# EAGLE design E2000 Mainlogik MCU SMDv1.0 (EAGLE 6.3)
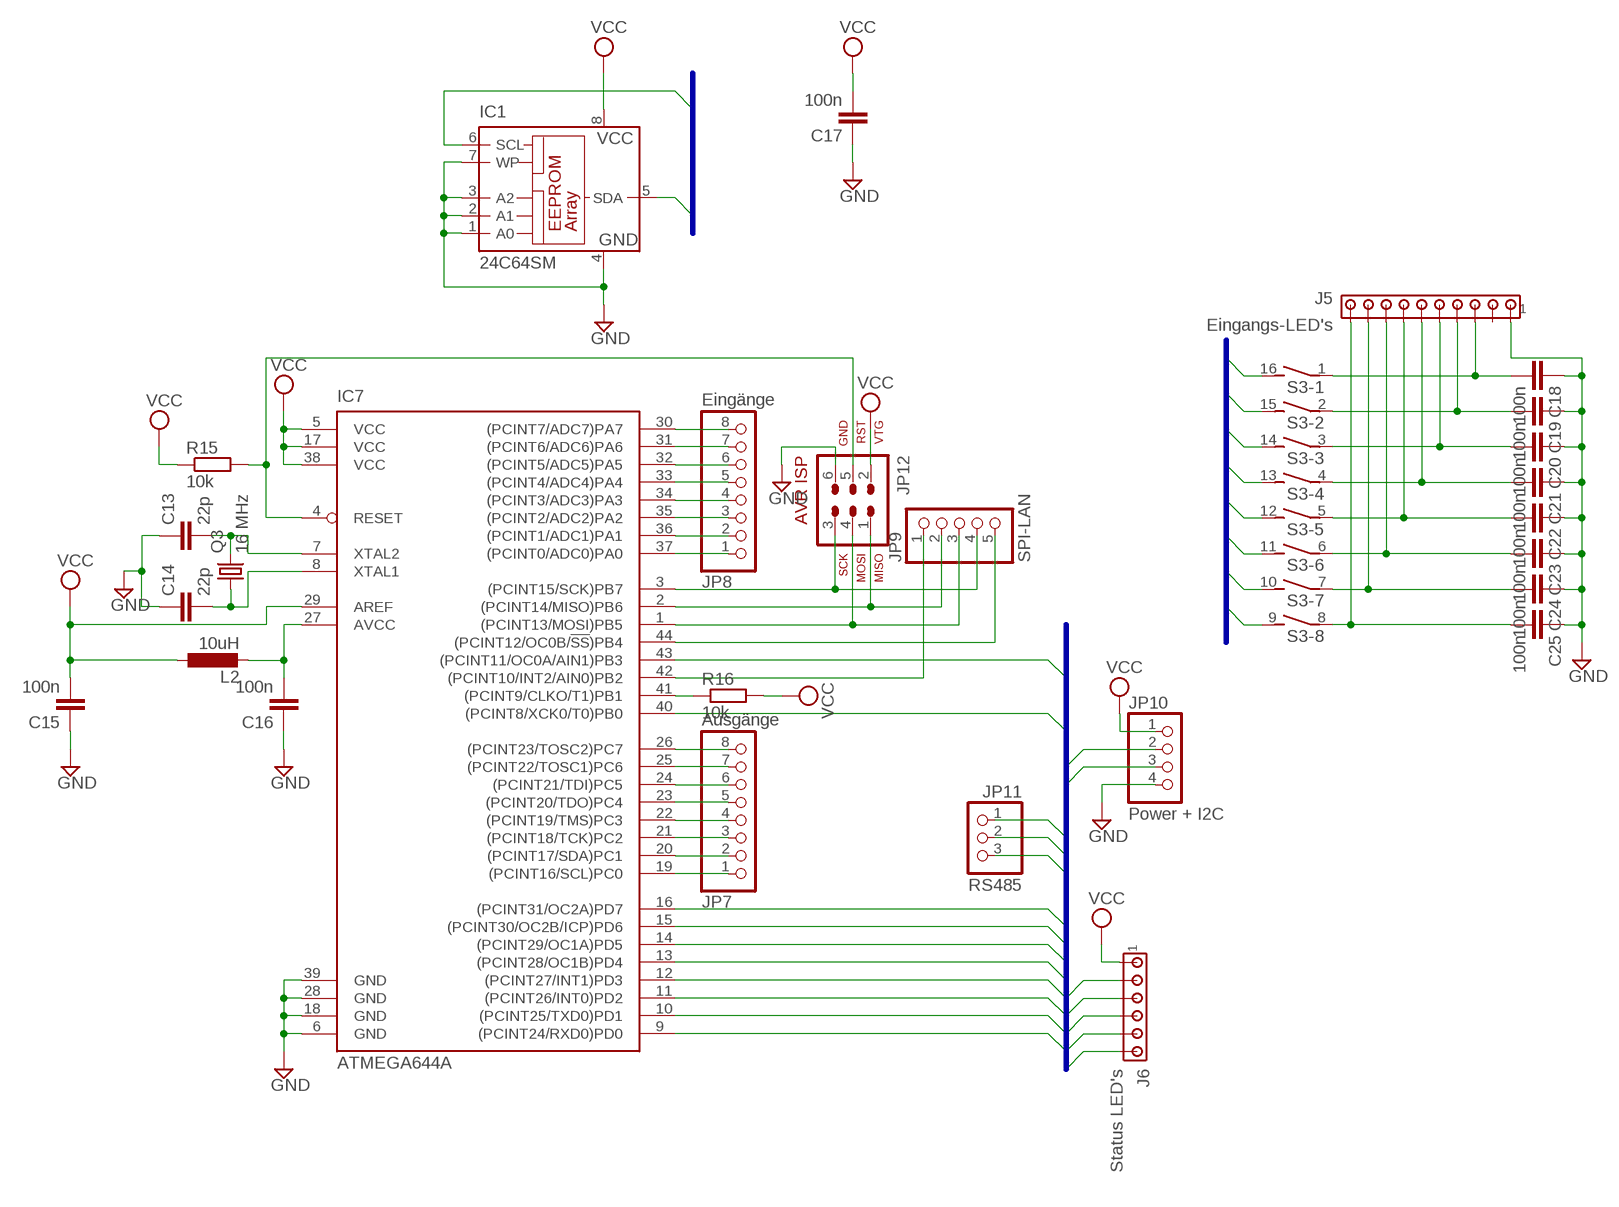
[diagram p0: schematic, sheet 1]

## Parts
C13  22p  C-EUC1206  [C1206]
C14  22p  C-EUC1206  [C1206]
C15  100n  C-EUC1206  [C1206]
C16  100n  C-EUC1206  [C1206]
C17  100n  C-EUC1206  [C1206]
C18  100n  C-EUC1206  [C1206]
C19  100n  C-EUC1206  [C1206]
C20  100n  C-EUC1206  [C1206]
C21  100n  C-EUC1206  [C1206]
C22  100n  C-EUC1206  [C1206]
C23  100n  C-EUC1206  [C1206]
C24  100n  C-EUC1206  [C1206]
C25  100n  C-EUC1206  [C1206]
IC1  24C64SM  [SO-08M]
IC7  ATMEGA644A  [TQFP44]
J5  Eingangs-LED's  MTA10-100  [10X10MTA]
J6  Status LED's  MTA06-100  [10X06MTA]
JP7  Ausgänge  PINHD-1X8_2.54-SMD  [1X08SMD]
JP8  Eingänge  PINHD-1X8_2.54-SMD  [1X08SMD]
JP9  SPI-LAN  PINHD-1X5_2.54-SMD  [1X05SMD]
JP10  Power + I2C  PINHD-1X4_2.54-SMD  [1X04SMD]
JP11  RS485  PINHD-1X3_2.54-SMD  [1X03SMD]
JP12  AVR-ISP-6  [AVR-ISP-6]
L2  10uH  L-EUL1206  [C1206]
Q3  16 MHz  CRYSTALHC49S  [HC49/S]
R15  10k  R-EU_0207/10  [0207/10]
R16  10k  R-EU_0207/10  [0207/10]
S3  DIP08S  [DIP08S]

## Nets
A1: IC7.19((PCINT16/SCL)PC0) JP7.1
A2: IC7.20((PCINT17/SDA)PC1) JP7.2
A3: IC7.21((PCINT18/TCK)PC2) JP7.3
A4: IC7.22((PCINT19/TMS)PC3) JP7.4
A5: IC7.23((PCINT20/TDO)PC4) JP7.5
A6: IC7.24((PCINT21/TDI)PC5) JP7.6
A7: IC7.25((PCINT22/TOSC1)PC6) JP7.7
A8: IC7.26((PCINT23/TOSC2)PC7) JP7.8
CS: IC7.44((PCINT12/OC0B/!SS!)PB4) JP9.5
E1: IC7.37((PCINT0/ADC0)PA0) JP8.1 S3.16
E2: IC7.36((PCINT1/ADC1)PA1) JP8.2 S3.15
E3: IC7.35((PCINT2/ADC2)PA2) JP8.3 S3.14
E4: IC7.34((PCINT3/ADC3)PA3) JP8.4 S3.13
E5: IC7.33((PCINT4/ADC4)PA4) JP8.5 S3.12
E6: IC7.32((PCINT5/ADC5)PA5) JP8.6 S3.11
E7: IC7.31((PCINT6/ADC6)PA6) JP8.7 S3.10
E8: IC7.30((PCINT7/ADC7)PA7) JP8.8 S3.9
EXT3: IC7.13((PCINT28/OC1B)PD4) JP11.2
EXT4: IC7.14((PCINT29/OC1A)PD5) J6.1
EXT5: IC7.15((PCINT30/OC2B/ICP)PD6) J6.2
EXT6: IC7.16((PCINT31/OC2A)PD7) J6.3
EXT7: IC7.40((PCINT8/XCK0/T0)PB0) J6.4
EXT8: IC7.43((PCINT11/OC0A/AIN1)PB3) J6.5
GND: C13.1 C14.1 C15.1 C16.1 C17.1 C18.1 C19.1 C20.1 C21.1 C22.1 C23.1 C24.1 C25.1 IC1.1(A0) IC1.2(A1) IC1.3(A2) IC1.4(GND) IC1.7(WP) IC7.6(GND) IC7.18(GND) IC7.28(GND) IC7.39(GND) J5.1 JP10.4 JP12.6
INT: IC7.42((PCINT10/INT2/AIN0)PB2) JP9.1
MISO: IC7.2((PCINT14/MISO)PB6) JP9.2 JP12.1
MOSI: IC7.1((PCINT13/MOSI)PB5) JP9.3 JP12.4
N$1: C18.2 J5.3 S3.1
N$2: C19.2 J5.4 S3.2
N$3: IC7.41((PCINT9/CLKO/T1)PB1) R16.1
N$4: C20.2 J5.5 S3.3
N$5: C21.2 J5.6 S3.4
N$6: C22.2 J5.7 S3.5
N$7: C23.2 J5.8 S3.6
N$8: C24.2 J5.9 S3.7
N$9: C25.2 J5.10 S3.8
N$17: C14.2 IC7.8(XTAL1) Q3.1
N$18: C13.2 IC7.7(XTAL2) Q3.2
N$19: C16.2 IC7.27(AVCC) L2.2
RST: IC7.4(RESET) JP12.5 R15.2
RX: IC7.9((PCINT24/RXD0)PD0) JP11.3
SCK: IC7.3((PCINT15/SCK)PB7) JP9.4 JP12.3
SCL: IC1.6(SCL) IC7.11((PCINT26/INT0)PD2) JP10.2
SDA: IC1.5(SDA) IC7.12((PCINT27/INT1)PD3) JP10.3
TX: IC7.10((PCINT25/TXD0)PD1) JP11.1
VCC: C15.2 C17.2 IC1.8(VCC) IC7.5(VCC) IC7.17(VCC) IC7.29(AREF) IC7.38(VCC) J6.6 JP10.1 JP12.2 L2.1 R15.1 R16.2
Unconnected: J5.2

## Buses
E1,E2,E3,E4,E5,E6,E7,E8
RX,TX,SCL,SDA,EXT3,EXT4,EXT5,EXT6,EXT7,EXT8
SCL,SDA

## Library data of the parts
C13-C25 = rcl:C-EU: CAPACITOR, European symbol
IC1 = microchip:24*: Serial EEPROM I2C; MF: RAMTRON INTERNATIONAL CORP; MPN: FM24C64-S; OC_FARNELL: 9882685; OC_NEWARK: 98H0189
IC7 = atmel:ATMEGA644: 8-bit Microcontroller with 64K Bytes In-System Programmable Flash Source: http://www.atmel.com/dyn/resources/prod_documents/doc2593.pdf; MPN: ATMEGA644PV-10AU; OC_FARNELL: 1455123; OC_NEWARK: 58M3748
J5 = con-amp:MTA10-100: AMP connector
J6 = con-amp:MTA06-100: AMP connector
JP7 JP8 = pinhead:PINHD-1X8: PIN HEADER
JP9 = pinhead:PINHD-1X5: PIN HEADER
JP10 = pinhead:PINHD-1X4: PIN HEADER
JP11 = pinhead:PINHD-1X3: PIN HEADER
JP12 = avr-6:AVR-ISP-6: AVR ISP-6 Serial Programming Header
L2 = rcl:L-EU: INDUCTOR, European symbol
Q3 = crystal:CRYSTAL: CRYSTAL; OC_FARNELL: 1667008; OC_NEWARK: unknown
R15 R16 = rcl:R-EU_: RESISTOR, European symbol
S3 = switch-dil:DIP08S: DIL/CODE SWITCH; OC_FARNELL: unknown; OC_NEWARK: unknown

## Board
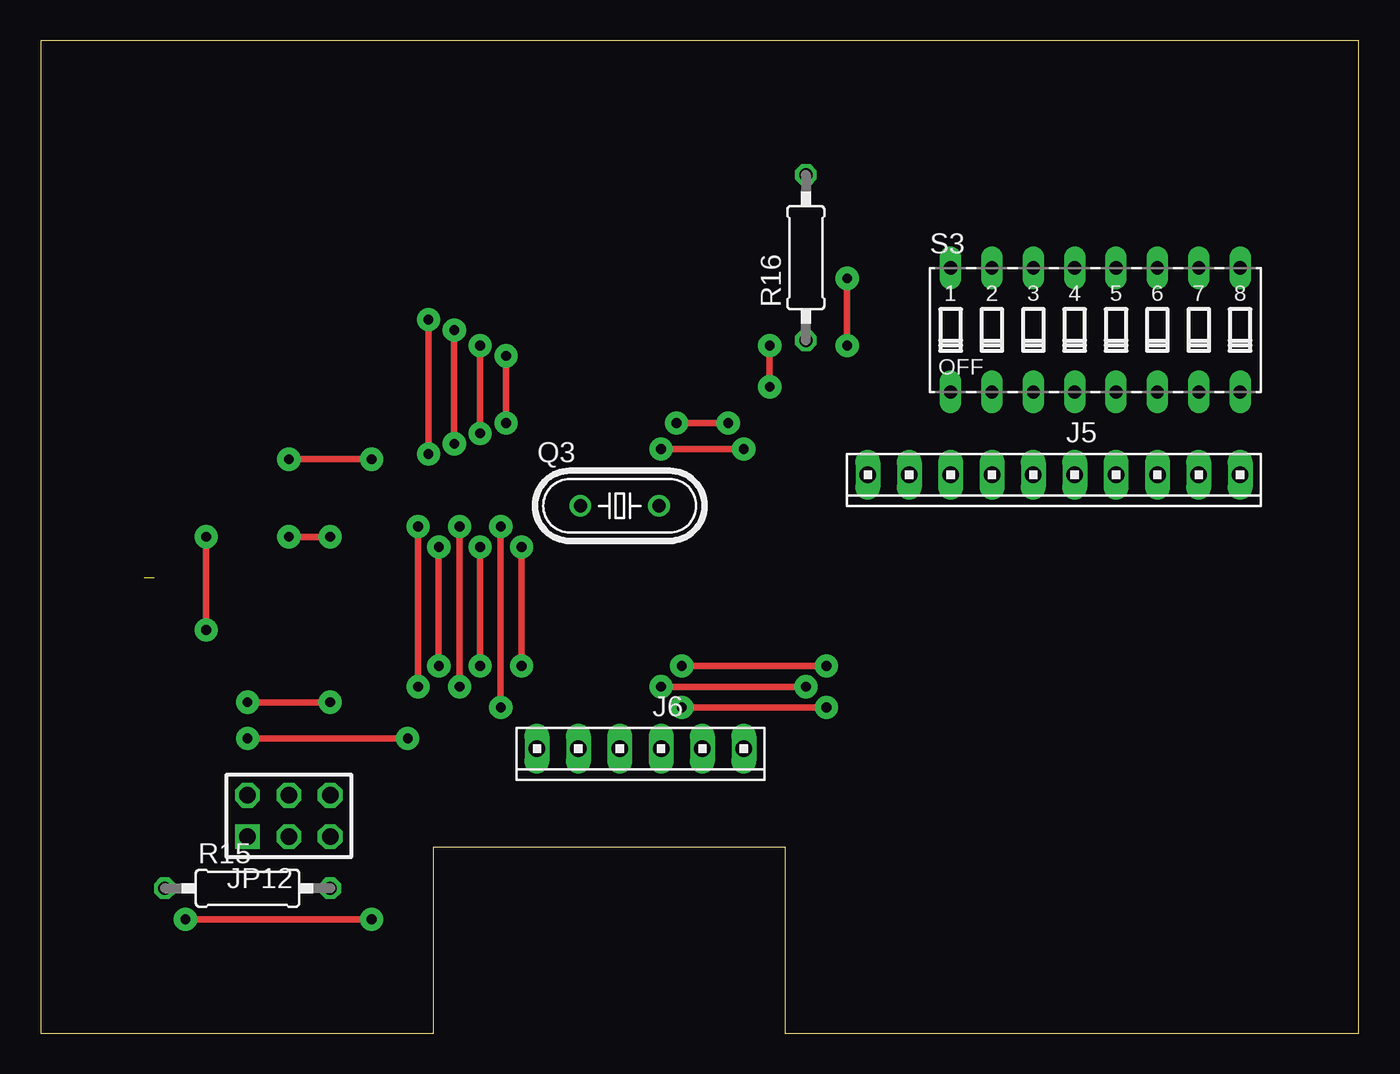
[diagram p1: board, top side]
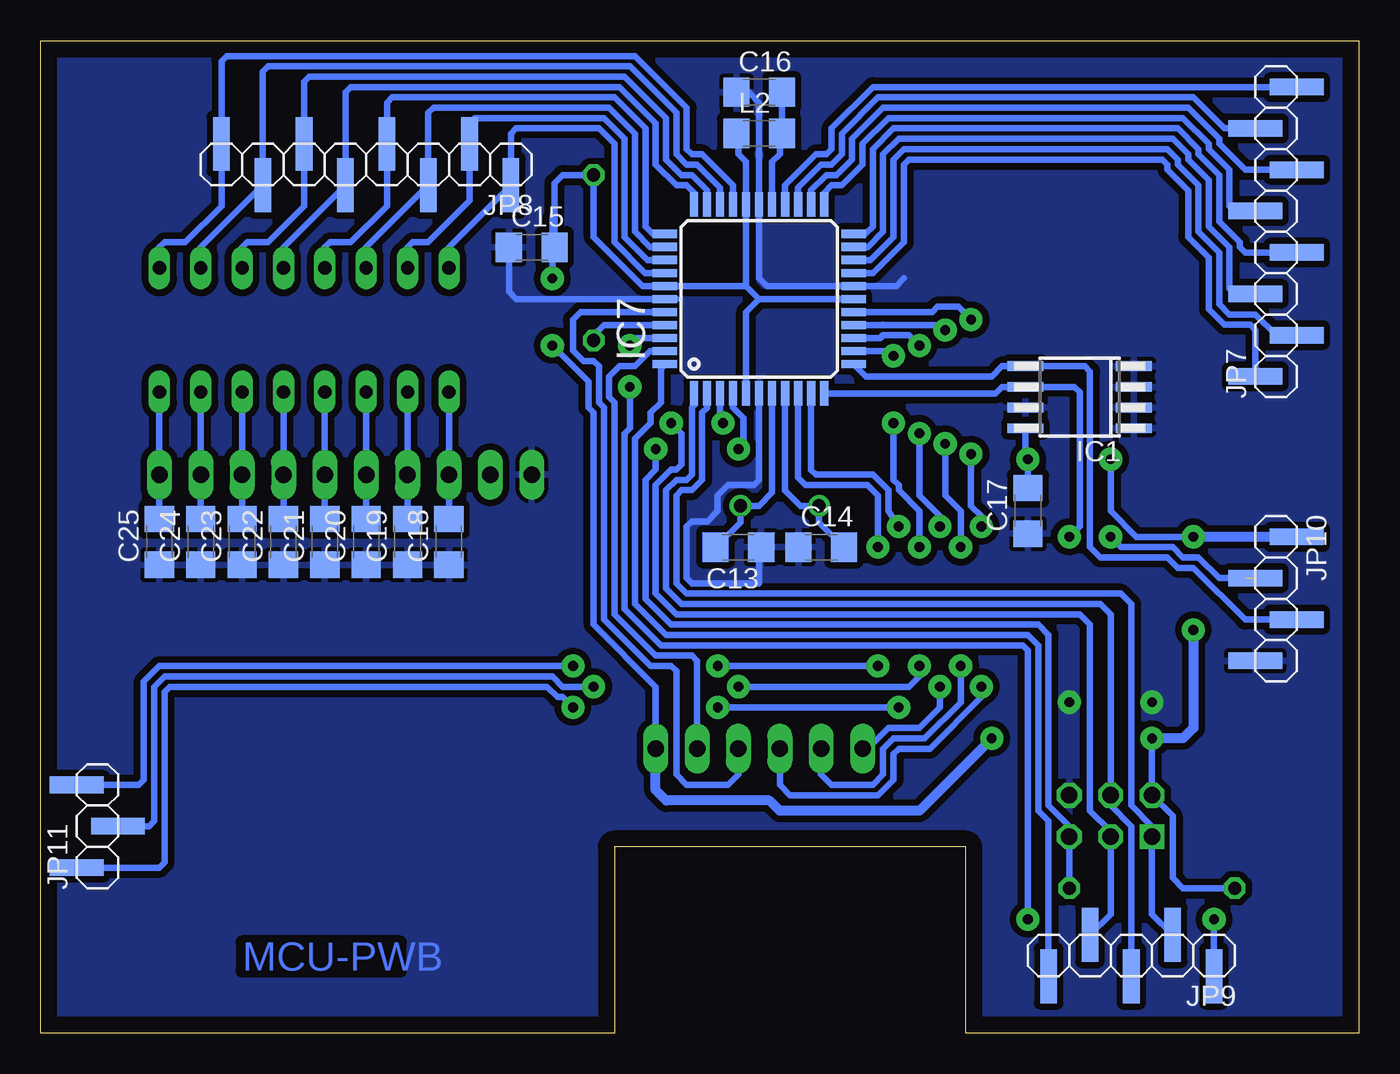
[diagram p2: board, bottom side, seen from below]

Size 80.95 x 60.95 mm. Coordinates in mm from the lower left corner, seen from the top.
Outline: 0,0 24.13,0 24.13,11.43 45.72,11.43 45.72,0 80.95,0 80.95,60.95 0,60.95 0,0
Copper layers (1*16): Top 0.035mm / dielectric 1.5mm / Bottom 0.035mm
Design rules "default": minimum track width 10mil, minimum drill 24mil, track to track 8mil, track to pad 8mil, pad to pad 8mil, via to via 8mil, smd to smd 8mil, copper to edge 40mil, drill to drill 8mil, minimum pad ring 10mil, minimum via ring 8mil, stop-mask expansion 4mil, vias tented up to drill 0mil, thermal gap 10mil

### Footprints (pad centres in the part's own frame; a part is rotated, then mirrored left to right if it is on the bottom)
C1206 = smd 1.6 x 1.8: 1 -1.4,0; 2 1.4,0
SO-08M = smd 0.6 x 2.2: 1 -1.905,-3.33; 2 -0.635,-3.33; 3 0.635,-3.33; 4 1.905,-3.33; 5 1.905,3.33; 6 0.635,3.33; 7 -0.635,3.33; 8 -1.905,3.33
TQFP44 = smd 1.5 x 0.5: 1 -5.8,4; 2 -5.8,3.2; 3 -5.8,2.4; 4 -5.8,1.6; 5 -5.8,0.8; 6 -5.8,0; 7 -5.8,-0.8; 8 -5.8,-1.6; 9 -5.8,-2.4; 10 -5.8,-3.2; 11 -5.8,-4; 23 5.8,-4; 24 5.8,-3.2; 25 5.8,-2.4; 26 5.8,-1.6; 27 5.8,-0.8; 28 5.8,0; 29 5.8,0.8; 30 5.8,1.6; 31 5.8,2.4; 32 5.8,3.2; 33 5.8,4 | smd 0.5 x 1.5: 12 -4,-5.8; 13 -3.2,-5.8; 14 -2.4,-5.8; 15 -1.6,-5.8; 16 -0.8,-5.8; 17 0,-5.8; 18 0.8,-5.8; 19 1.6,-5.8; 20 2.4,-5.8; 21 3.2,-5.8; 22 4,-5.8; 34 4,5.8; 35 3.2,5.8; 36 2.4,5.8; 37 1.6,5.8; 38 0.8,5.8; 39 0,5.8; 40 -0.8,5.8; 41 -1.6,5.8; 42 -2.4,5.8; 43 -3.2,5.8; 44 -4,5.8
10X10MTA = drill 1.016 long: 1 11.43,0; 2 8.89,0; 3 6.35,0; 4 3.81,0; 5 1.27,0; 6 -1.27,0; 7 -3.81,0; 8 -6.35,0; 9 -8.89,0; 10 -11.43,0
10X06MTA = drill 1.016 long: 1 6.35,0; 2 3.81,0; 3 1.27,0; 4 -1.27,0; 5 -3.81,0; 6 -6.35,0
1X08SMD = smd 1.016 x 3.302: 1 -1.27,1.27; 2 1.27,-1.27; 3 3.81,1.27; 4 6.35,-1.27; 5 8.89,1.27; 6 11.43,-1.27; 7 13.97,1.27; 8 16.51,-1.27
1X05SMD = smd 1.016 x 3.302: 1 -1.27,1.27; 2 1.27,-1.27; 3 3.81,1.27; 4 6.35,-1.27; 5 8.89,1.27
1X04SMD = smd 1.016 x 3.302: 1 -1.27,1.27; 2 1.27,-1.27; 3 3.81,1.27; 4 6.35,-1.27
1X03SMD = smd 1.016 x 3.302: 1 -1.27,1.27; 2 1.27,-1.27; 3 3.81,1.27
AVR-ISP-6 = drill 1.016 square: 1 -2.54,-1.27 | drill 1.016 octagon: 2 -2.54,1.27; 3 0,-1.27; 4 0,1.27; 5 2.54,-1.27; 6 2.54,1.27
HC49/S = drill 0.813: 1 -2.413,0; 2 2.413,0
0207/10 = drill 0.813 octagon: 1 -5.08,0; 2 5.08,0
DIP08S = drill 0.813 long: 1 -8.89,-3.81; 2 -6.35,-3.81; 3 -3.81,-3.81; 4 -1.27,-3.81; 5 1.27,-3.81; 6 3.81,-3.81; 7 6.35,-3.81; 8 8.89,-3.81; 9 8.89,3.81; 10 6.35,3.81; 11 3.81,3.81; 12 1.27,3.81; 13 -1.27,3.81; 14 -3.81,3.81; 15 -6.35,3.81; 16 -8.89,3.81

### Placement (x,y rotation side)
C13  38.1,29.84 180 bottom
C14  33.02,29.84 0 bottom
C15  50.8,48.26 0 bottom
C16  36.83,57.78 0 bottom
C17  20.32,32.07 90 bottom
C18  55.88,30.16 90 bottom
C19  58.42,30.16 90 bottom
C20  60.96,30.16 90 bottom
C21  63.5,30.16 90 bottom
C22  66.04,30.16 90 bottom
C23  68.58,30.16 90 bottom
C24  71.12,30.16 90 bottom
C25  73.66,30.16 90 bottom
IC1  17.14,39.05 90 bottom
IC7  36.83,45.09 90 bottom
J5  62.23,34.29 180 top
J6  36.83,17.46 180 top
JP7  5.08,41.59 90 bottom
JP8  53.34,53.34 180 bottom
JP9  10.16,4.76 180 bottom
JP10  5.08,29.21 270 bottom
JP11  77.47,11.43 90 bottom
JP12  15.24,13.34 0 top
L2  36.83,55.24 0 bottom
Q3  35.56,32.38 0 top
R15  12.7,8.89 0 top
R16  46.99,47.62 90 top
S3  64.77,43.18 0 top

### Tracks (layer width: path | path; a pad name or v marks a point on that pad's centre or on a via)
A1
  Bottom 0.406: IC7.19 29.83,46.69 27.94,48.58 27.94,53.34 27.62,53.66 12.07,53.66 11.75,53.34 11.75,53.02 10.48,51.75 10.48,48.9 9.21,47.62 9.21,44.45 8.26,43.5 6.67,43.5 6.35,43.18 JP7.1
A2
  Bottom 0.406: IC7.20 29.98,47.48 28.57,48.9 28.57,53.66 27.94,54.29 11.75,54.29 11.11,53.66 11.11,53.34 9.84,52.07 9.84,49.21 8.57,47.94 8.57,44.77 7.94,44.13 6.35,44.13 5.08,42.86 JP7.2
A3
  Bottom 0.406: IC7.21 30.14,48.28 29.21,49.21 29.21,53.98 28.26,54.93 11.43,54.93 10.48,53.98 10.48,53.66 9.21,52.39 9.21,49.53 7.94,48.26 7.94,45.72 7.62,45.4 JP7.3
A4
  Bottom 0.406: IC7.22 30.29,49.09 29.84,49.53 29.84,54.29 28.57,55.56 11.11,55.56 9.84,54.29 9.84,53.98 8.57,52.7 8.57,49.85 7.3,48.58 7.3,48.26 6.99,47.94 JP7.4
A5
  Bottom 0.406: IC7.23 32.83,51.62 32.38,52.07 31.75,52.07 30.48,53.34 30.48,54.61 28.89,56.2 10.79,56.2 9.21,54.61 9.21,54.29 7.94,53.02 7.94,50.8 7.62,50.48 JP7.5
A6
  Bottom 0.406: IC7.24 33.63,51.78 32.7,52.7 32.07,52.7 31.11,53.66 31.11,54.93 29.21,56.83 10.48,56.83 8.57,54.93 8.57,54.61 6.99,53.02 JP7.6
A7
  Bottom 0.406: IC7.25 34.43,51.93 33.02,53.34 32.38,53.34 31.75,53.98 31.75,55.24 29.53,57.47 10.16,57.47 8.26,55.56 JP7.7
A8
  Bottom 0.406: IC7.26 35.23,52.08 33.34,53.98 32.7,53.98 32.38,54.29 32.38,55.56 29.84,58.1 JP7.8
CS
  Bottom 0.406: IC7.44 42.86,40.85 42.86,38.73 43.5,38.1 43.5,37.47 44.45,36.51 44.45,26.35 42.54,24.45 20.32,24.45 19.68,23.81 19.68,13.65 19.05,13.02 JP9.5
E1
  Bottom 0.406: IC7.37 43.83,46.69 45.72,48.58 45.72,54.61 46.67,55.56 51.75,55.56 52.07,55.24 JP8.1 55.88,48.26 S3.16
E2
  Bottom 0.406: IC7.36 43.67,47.48 45.08,48.9 45.08,54.93 46.35,56.2 54.29,56.2 54.61,55.88 JP8.2 54.61,51.12 57.15,48.58 58.1,48.58 58.42,48.26 S3.15
E3
  Bottom 0.406: IC7.35 43.52,48.28 44.45,49.21 44.45,55.24 46.04,56.83 56.83,56.83 57.15,56.52 JP8.3 60.96,48.26 S3.14
E4
  Bottom 0.406: IC7.34 43.37,49.09 43.81,49.53 43.81,55.56 45.72,57.47 59.37,57.47 59.69,57.15 JP8.4 59.69,50.8 61.91,48.58 63.18,48.58 63.5,48.26 S3.13
E5
  Bottom 0.406: IC7.33 40.83,51.62 41.27,52.07 41.91,52.07 43.18,53.34 43.18,55.88 45.4,58.1 61.91,58.1 62.23,57.78 JP8.5 66.04,48.26 S3.12
E6
  Bottom 0.406: IC7.32 40.03,51.78 40.96,52.7 41.59,52.7 42.54,53.66 42.54,56.2 45.08,58.74 64.45,58.74 64.77,58.42 JP8.6 64.77,50.8 66.99,48.58 68.26,48.58 68.58,48.26 S3.11
E7
  Bottom 0.406: IC7.31 39.23,51.93 40.64,53.34 41.27,53.34 41.91,53.98 41.91,56.52 44.77,59.37 66.99,59.37 67.31,59.05 JP8.7 71.12,48.26 S3.10
E8
  Bottom 0.406: IC7.30 38.43,52.08 40.32,53.98 40.96,53.98 41.27,54.29 41.27,56.83 44.45,60.01 69.53,60.01 69.85,59.69 JP8.8 69.85,50.8 72.07,48.58 73.34,48.58 73.66,48.26 S3.9
EXT3  (via drill 0.6 pad 1.42)
  Top 0.406: v28.57,41.59 v28.57,37.47 | v46.99,21.27 v38.1,21.27 | v26.99,22.54 v26.99,29.84
  Bottom 0.406: IC7.13 28.87,41.88 v28.57,41.59 | v46.99,21.27 48.89,21.27 49.53,21.91 73.34,21.91 73.98,21.27 73.98,13.02 74.3,12.7 JP11.2 | v38.1,21.27 27.62,21.27 26.99,21.91 v26.99,22.54 | v26.99,29.84 26.99,32.07 28.26,33.34 28.26,33.66 28.57,33.97 v28.57,37.47
EXT4  (via drill 0.6 pad 1.42)
  Top 0.406: v26.99,42.23 v26.99,36.83 | v25.72,31.11 v25.72,21.27
  Bottom 0.406: v26.99,42.23 27.62,42.86 29.21,42.86 29.39,42.69 IC7.14 | v26.99,36.83 26.99,33.02 25.72,31.75 v25.72,31.11 | v25.72,21.27 25.72,20 26.99,18.73 28.89,18.73 30.16,17.46 J6.1
EXT5  (via drill 0.6 pad 1.42)
  Top 0.406: v25.4,43.18 v25.4,36.2 | v24.45,29.84 v24.45,22.54
  Bottom 0.406: v25.4,43.18 25.71,43.48 29.2,43.48 29.21,43.5 29.22,43.48 IC7.15 | v25.4,36.2 25.4,33.02 24.45,32.07 v24.45,29.84 | v24.45,22.54 24.45,20.32 26.67,18.1 28.57,18.1 29.21,17.46 29.21,15.88 29.84,15.24 32.38,15.24 33.02,15.88 J6.2
EXT6  (via drill 0.6 pad 1.42)
  Top 0.406: v23.81,43.81 v23.81,35.56 | v23.18,31.11 v23.18,21.27
  Bottom 0.406: v23.81,43.81 24.6,44.6 25.88,44.6 26.2,44.28 IC7.16 | v23.81,35.56 23.81,32.38 23.18,31.75 v23.18,31.11 | v23.18,21.27 23.18,20.64 26.35,17.46 28.26,17.46 28.57,17.14 28.57,15.56 29.53,14.61 34.92,14.61 35.56,15.24 J6.3
EXT7
  Bottom 0.406: IC7.40 47.79,44.28 48.26,43.81 48.26,41.91 47.62,41.27 46.99,41.27 46.67,40.96 46.67,38.73 46.35,38.42 46.35,25.4 43.5,22.54 42.23,22.54 41.91,22.23 41.91,15.88 41.27,15.24 38.73,15.24 38.1,15.88 J6.4
EXT8
  Bottom 0.406: IC7.43 43.52,41.88 44.45,40.96 45.4,40.96 46.04,40.32 46.04,39.05 45.72,38.73 45.72,25.72 43.18,23.18 40.96,23.18 40.64,22.86 J6.5
GND  (via drill 0.6 pad 1.42)
  Top 0.406: v17.78,20.32 v12.7,20.32
  Bottom 0.406: 37.46,57.78 36.83,57.15 IC7.28 36.83,46.35 36.36,45.88 IC7.18 28.41,45.88 27.94,46.35 | 41.91,45.09 IC7.39 51.75,45.09 52.2,45.53 C15.1 | IC7.6 36.83,33.97 37.15,33.66 38.73,33.66 39.37,33.02 39.37,32.07 40,31.43 40.96,31.43 41.27,31.11 41.27,27.94 40.96,27.62 36.83,27.62 36.83,29.71 C13.1
  pour Bottom (isolate 0.406): -1.27,62.23 82.55,62.23 82.55,-1.27 44.45,-1.27 44.45,10.16 25.4,10.16 25.4,-1.27 -1.27,-1.27
INT  (via drill 0.6 pad 1.42)
  Top 0.406: v44.77,42.23 v44.77,39.69 | v8.89,6.99 v20.32,6.99
  Bottom 0.406: v20.32,6.99 20.32,23.5 20.64,23.81 42.86,23.81 45.08,26.04 45.08,36.83 44.77,37.15 v44.77,39.69 | IC7.42 44.31,42.69 v44.77,42.23 | JP9.1 v8.89,6.99
MISO
  Bottom 0.406: IC7.2 40.03,38.39 40.32,38.1 40.32,33.97 40.96,33.34 41.59,33.34 41.91,33.02 41.91,27.62 41.27,26.99 14.61,26.99 13.97,26.35 13.97,13.97 12.7,12.7 JP12.1 12.7,7.3 JP9.2
MOSI
  Bottom 0.406: IC7.1 40.83,38.55 40.96,38.42 40.96,34.29 41.27,33.97 41.91,33.97 42.54,33.34 42.54,27.3 41.59,26.35 15.88,26.35 15.24,25.72 JP12.4 15.24,13.97 13.97,12.7 JP9.3
N$1
  Bottom 0.406: C18.2 J5.3 S3.1
N$2
  Bottom 0.406: C19.2 J5.4 S3.2
N$3
  Bottom 0.406: IC7.41 46.37,43.48 46.99,42.86 R16.1
N$4
  Bottom 0.406: C20.2 J5.5 S3.3
N$5
  Bottom 0.406: C21.2 J5.6 S3.4
N$6
  Bottom 0.406: C22.2 J5.7 S3.5
N$7
  Bottom 0.406: C23.2 J5.8 S3.6
N$8
  Bottom 0.406: S3.7 J5.9 C24.2
N$9
  Bottom 0.406: C25.2 J5.10 S3.8
N$17
  Bottom 0.406: IC7.8 35.23,33.33 34.29,32.38 Q3.1 33.15,31.37 C14.2
N$18
  Bottom 0.406: IC7.7 36.03,33.19 36.83,32.38 Q3.2 37.97,31.37 C13.2
N$19
  Bottom 0.406: IC7.27 36.03,53.51 35.56,53.98 35.56,55.12 L2.2 C16.2
RST  (via drill 0.6 pad 1.42)
  Top 0.406: v38.1,35.88 v43.18,35.88
  Bottom 0.406: R15.2 JP12.5 17.78,12.7 19.05,13.97 19.05,24.45 19.68,25.08 42.23,25.08 43.81,26.67 43.81,33.97 43.18,34.61 v43.18,35.88 | IC7.4 38.43,38.43 37.78,37.78 37.78,36.2 v38.1,35.88
RX  (via drill 0.6 pad 1.42)
  Top 0.406: v29.53,29.84 v29.53,22.54 | v48.26,22.54 v39.37,22.54
  Bottom 0.406: IC7.9 34.43,34.11 33.97,33.66 30.16,33.66 29.53,33.02 v29.53,29.84 | v48.26,22.54 73.66,22.54 74.61,21.59 74.61,15.56 74.93,15.24 JP11.3 | v39.37,22.54 v29.53,22.54
SCK  (via drill 0.6 pad 1.42)
  Top 0.406: v39.05,37.47 v42.23,37.47
  Bottom 0.406: IC7.3 39.23,37.6 v39.05,37.47 | v42.23,37.47 41.59,36.83 41.59,34.92 41.91,34.61 42.23,34.61 43.18,33.66 43.18,26.99 41.91,25.72 17.14,25.72 16.51,25.08 16.51,13.65 15.24,12.38 JP12.3 15.24,7.3 JP9.4
SCL  (via drill 0.6 pad 1.42)  (1 unrouted)
  Top 0.406: v15.24,30.48 v17.78,30.48
  Bottom 0.406: IC7.11 22.31,39.28 21.91,39.69 IC1.6 17.46,39.69 17.14,39.37 17.14,31.11 v17.78,30.48 | 7.3,27.62 6.99,27.94 | JP10.2 8.57,27.94 9.84,29.21 10.79,29.21 11.43,29.84 14.61,29.84 v15.24,30.48
SDA
  Bottom 0.406: IC7.12 30.27,40.32 22.54,40.32 21.91,40.96 IC1.5 16.83,40.96 16.51,40.64 16.51,29.84 15.88,29.21 11.75,29.21 11.11,28.57 10.16,28.57 6.99,25.4 JP10.3
TX  (via drill 0.6 pad 1.42)
  Top 0.406: v48.26,20 v39.37,20 | v28.26,20 v28.26,31.11
  Bottom 0.406: IC7.10 33.63,34.58 33.34,34.29 29.84,34.29 28.89,33.34 28.89,32.07 v28.26,31.11 | v48.26,20 48.89,20.64 49.21,20.64 49.85,21.27 73.03,21.27 73.34,20.95 73.34,10.48 73.66,10.16 JP11.1 | v39.37,20 v28.26,20
VCC  (via drill 0.6 pad 1.42)
  Top 0.406: v49.53,42.23 v49.53,46.35 | v12.7,18.1 v22.54,18.1 | v10.16,24.77 v10.16,30.48 | v20.32,35.24 v15.24,35.24
  Bottom 0.406: IC7.17 36.83,45.09 | 37.63,45.88 IC7.38 43.98,45.88 46.99,48.9 R16.2 48.89,52.7 49.4,52.2 C15.2 49.53,50.03 v49.53,46.35 | 37.63,45.88 36.83,45.09 | IC7.5 37.63,44.28 36.83,45.09 | 37.63,45.88 IC7.29 37.63,53.51 38.1,53.98 38.1,55.12 L2.1 38.26,55.21 | R15.1 10.79,8.89 11.43,9.53 11.43,13.34 JP12.2 v12.7,18.1 | J6.6 43.18,21.27 46.99,25.08 46.99,38.1 47.31,38.42 47.31,40.01 v49.53,42.23 | IC1.8 20.48,35.4 v20.32,35.24 C17.2 | v15.24,35.24 15.24,32.07 13.65,30.48 v10.16,30.48
  Bottom 0.61: v10.16,24.77 10.16,18.73 10.79,18.1 v12.7,18.1 | v22.54,18.1 26.99,13.65 35.56,13.65 36.2,14.29 42.54,14.29 43.18,14.92 J6.6 | JP10.1 v10.16,30.48

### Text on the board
Bottom: MCU-PWB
